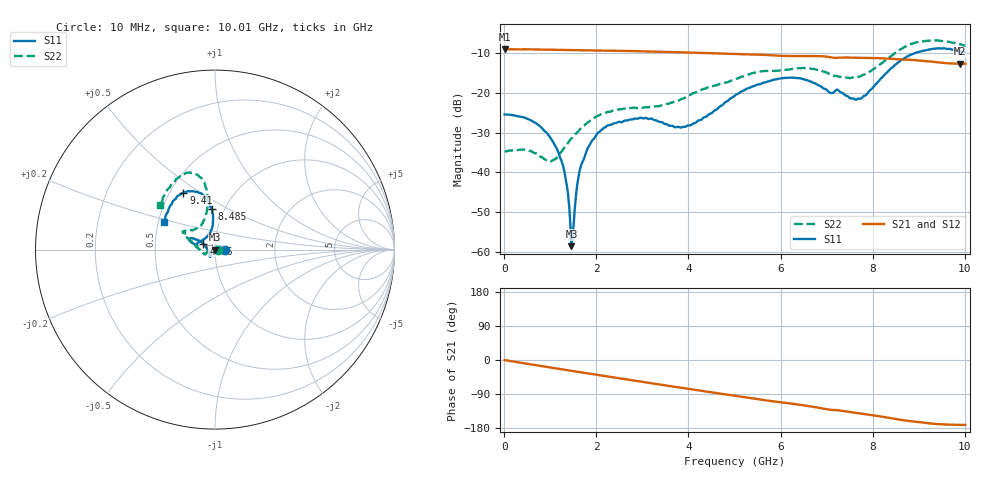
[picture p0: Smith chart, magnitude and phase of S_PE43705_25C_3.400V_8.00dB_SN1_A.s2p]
! Device ID: PE43705
! Serial: 1
! Insertion: A
! Impedance: 50 ohm
! Temp: 25C
! VDD: 3.400V
! Attenuation Step: 8.00dB
#  Hz  S  RI  R  50
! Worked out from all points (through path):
!   401 points, 10 MHz to 10.01 GHz, reference 50 ohm
!   highest |S21| = -8.98 dB at 10 MHz (marker M1); lowest = -12.7 dB at 9.885 GHz (marker M2)
!   group delay of S21, straight-line fit = 49.4 ps
!   lowest |S11| = -58.5 dB at 1.46 GHz (marker M3), VSWR 1.00, Z = 50.1 - j0.0604 ohm
!   |S11| at or under -10 dB: start of sweep to 8.909 GHz
!   |S22| runs from -37.2 to -6.8 dB; largest |S21 - S12| = 0.0031
!   S11 on the Smith chart (normalised r, x): 10 MHz: 1.11, +0.00; 4.76 GHz: 0.88, +0.06; 8.485 GHz: 0.87, +0.41; 9.41 GHz: 0.59, +0.43; 10.01 GHz: 0.53, +0.19
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1e7  0.0537 4.03e-05  0.3554 -0.00162  0.3558 -0.00141  0.0184 0.000147
6.35e8  0.0404 0.0154  0.3433 -0.0767  0.3432 -0.0766  0.0087 0.0155
1.06e9  0.0211 0.0121  0.326 -0.1245  0.3262 -0.1244  -0.00828 0.0116
1.31e9  0.00861 0.00524  0.3135 -0.1505  0.3137 -0.1503  -0.02 0.0054
1.46e9  0.00102 -0.000603  0.3046 -0.1657  0.3048 -0.1657  -0.0268 0.000338
1.51e9  -0.000868 -0.00213  0.3014 -0.1707  0.3016 -0.1706  -0.0287 -0.00108
1.585e9  -0.00504 -0.00484  0.2965 -0.1777  0.2967 -0.1777  -0.0317 -0.00378
1.685e9  -0.00888 -0.00955  0.2901 -0.1871  0.29 -0.187  -0.0362 -0.00736
1.885e9  -0.0167 -0.0169  0.2757 -0.2051  0.2758 -0.2049  -0.0437 -0.0139
2.21e9  -0.0236 -0.0294  0.2501 -0.2318  0.2502 -0.2317  -0.0517 -0.0229
3.36e9  -0.028 -0.0334  0.1423 -0.2969  0.1427 -0.2965  -0.0659 -0.0176
3.985e9  -0.0383 -0.00646  0.078 -0.3128  0.0783 -0.3124  -0.0913 0.00446
4.76e9  -0.0643 0.0335  0.000512 -0.3117  0.000952 -0.3116  -0.1264 0.0415
5.01e9  -0.0809 0.0459  -0.0236 -0.3076  -0.0234 -0.3079  -0.1395 0.0522
5.985e9  -0.1379 0.0638  -0.1065 -0.2731  -0.1051 -0.2735  -0.1688 0.0901
6.685e9  -0.1305 0.0391  -0.159 -0.243  -0.1588 -0.243  -0.1716 0.1032
7.685e9  -0.0478 0.0703  -0.2131 -0.1767  -0.213 -0.1769  -0.0745 0.1418
8.36e9  -0.0114 0.1942  -0.2398 -0.1232  -0.2385 -0.1244  -0.0415 0.2781
8.485e9  -0.0186 0.2251  -0.2427 -0.1111  -0.2413 -0.1122  -0.0453 0.3147
9.41e9  -0.1757 0.3176  -0.2384 -0.0459  -0.2373 -0.0457  -0.1864 0.4168
9.885e9  -0.2677 0.2036  -0.2295 -0.0365  -0.2304 -0.0365  -0.2857 0.2975
1.001e10  -0.2845 0.1553  -0.2308 -0.0357  -0.2314 -0.0373  -0.3051 0.2488
